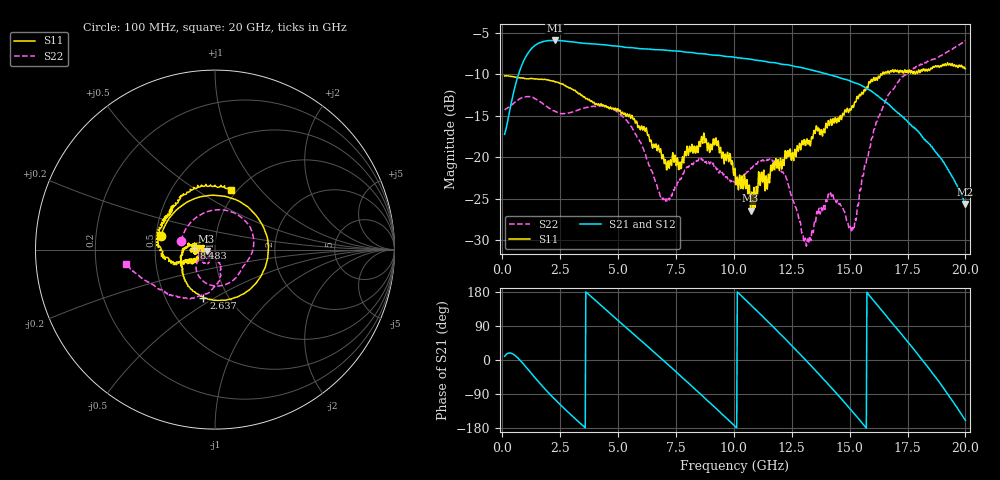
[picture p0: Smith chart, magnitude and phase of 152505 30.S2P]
!  2-Port S-parameters saved by WinCal
! VAR MeasName=S-Parameters (CALIBRATED_DATA) read from VNA (N5230C)
! VAR MeasDate=4/10/2015 9:31:19 AM
! VAR NAME=152505 30
! VAR FILENAME=152505 30.S2P
! VAR DATE=4/10/2015 9:31:19 AM
! VAR PHYS_PORTS=1,2
# Hz S DB R 50
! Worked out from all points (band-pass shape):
!   801 points, 100 MHz to 20 GHz, reference 50 ohm
!   highest |S21| = -5.92 dB at 2.264 GHz (marker M1); lowest = -25.6 dB at 20 GHz (marker M2)
!   |S21| within 3 dB of the highest: 838.2 MHz to 12.43 GHz (11.59 GHz wide, 175 % of centre)
!   lowest |S11| = -26.4 dB at 10.72 GHz (marker M3), VSWR 1.10, Z = 45.5 - j0.684 ohm
!   |S11| at or under -10 dB: start of sweep to 16.34 GHz; 16.37022 GHz to 16.41067 GHz (40.45 MHz wide, 0.247 % of centre)
!   |S22| runs from -30.7 to -6.0 dB; largest |S21 - S12| = 0.0067
!   S11 on the Smith chart (normalised r, x): 100 MHz: 0.53, +0.09; 2.637 GHz: 0.77, -0.44; 8.483 GHz: 0.79, +0.01; 20 GHz: 0.94, +0.70
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1e8  -10.19 166.2  -17.24 9.7  -17.21 9.6  -14.28 165.7
6.4725e8  -10.39 89.8  -10.48 6.7  -10.48 6.6  -13.16 91.9
1.219375e9  -10.49 14.5  -7.05 -32.6  -7.06 -32.6  -12.69 35.1
2.264125e9  -10.90 -81.4  -5.92 -103.5  -5.91 -103.4  -14.44 -21.7
2.63725e9  -11.20 -103.5  -5.99 -125.9  -6.00 -125.8  -14.73 -31.7
3.43325e9  -12.52 -136.7  -6.24 -170.7  -6.24 -170.6  -14.15 -54.5
4.1795e9  -13.60 -153.2  -6.40 148.8  -6.39 148.8  -13.82 -80.4
5.099875e9  -14.39 -170.2  -6.66 98.8  -6.70 98.5  -14.86 -116.2
6.741625e9  -18.54 166.5  -7.05 10.6  -7.04 10.4  -24.04 -147.7
7.51275e9  -21.00 -171.8  -7.19 -31.7  -7.20 -31.8  -23.52 -114.8
8.482875e9  -18.48 176.1  -7.50 -86.0  -7.44 -85.9  -20.21 -129.2
1.005e10  -21.33 169.3  -7.95 -174.9  -7.97 -175.0  -23.06 -140.1
1.072162e10  -26.44 -170.9  -8.17 145.6  -8.21 145.9  -21.39 -141.3
1.189075e10  -20.58 -154.3  -8.66 75.8  -8.66 75.8  -21.08 -170.0
1.3035e10  -17.87 -150.0  -9.29 4.2  -9.26 3.8  -30.27 -161.4
1.338325e10  -17.68 -152.5  -9.51 -18.3  -9.46 -18.2  -28.66 -134.4
1.417925e10  -15.40 -155.8  -10.09 -70.8  -10.00 -71.5  -24.29 -131.6
1.517425e10  -13.94 -160.2  -10.98 -139.7  -10.92 -139.7  -28.75 -98.0
1.602e10  -10.57 -174.3  -12.20 157.8  -12.13 157.3  -17.08 -77.9
1.669162e10  -9.83 169.4  -13.63 108.4  -13.75 107.1  -12.42 -97.3
1.793538e10  -9.91 139.2  -16.80 15.4  -17.10 15.9  -9.01 -134.9
2e10  -9.33 74.8  -25.62 -159.4  -25.68 -158.4  -5.97 -170.6
